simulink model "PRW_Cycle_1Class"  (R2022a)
settings: Solver=VariableStepAuto  StartTime=0.0  StopTime=simtime  RelTol=1e-3
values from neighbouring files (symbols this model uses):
  GT = SOH_p01(data_length_finish,1)    [Data_preparation.m]    (also in SimulationCycle.m = 1)
libraries: neural x35

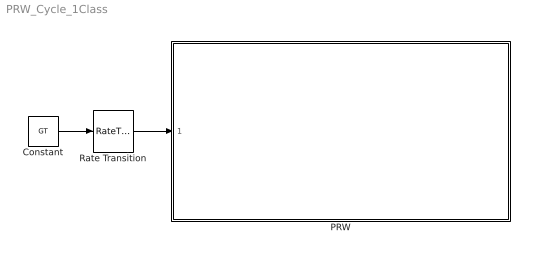
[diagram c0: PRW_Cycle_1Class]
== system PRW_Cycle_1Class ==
  Constant : Constant  Value=GT
  PRW : Subsystem
  Rate Transition : RateTransition  OutPortSampleTime=1
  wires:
  Rate Transition/1 -> PRW/1(SOH)
  Constant/1 -> Rate Transition/1

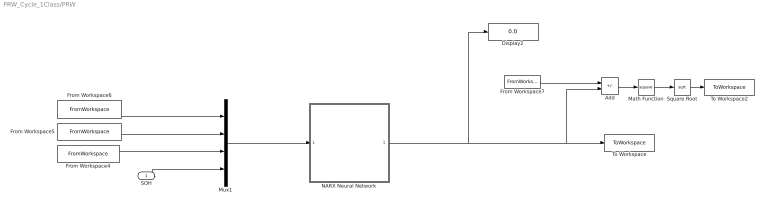
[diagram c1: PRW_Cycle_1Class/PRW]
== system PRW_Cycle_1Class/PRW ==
  SOH : Inport
  Add : Sum  Inputs=+-
  Display2 : Display
  From Workspace4 : FromWorkspace  VariableName=Temperature37
  From Workspace5 : FromWorkspace  VariableName=Voltage37  SampleTime=1
  From Workspace6 : FromWorkspace  VariableName=Current37  SampleTime=1
  From Workspace7 : FromWorkspace  VariableName=SOC_37_GT
  Math Function : Math  Operator=square
  Mux1 : Mux
  NARX Neural Network : Subsystem  mask{pi_input_1_delayed_1=[0.510586069346425031056924126460216939449310302734375;0.94022295872250705173200913122855126857757568359375;-0.58565072302558396355465220040059648454189300537109375;0.6993682659832136661037793601281009614467620849609375], ai_layer_2_delayed_1=0.999984478854660352453720406629145145416259765625}
      mask prompts: pi_input_1_delayed_1 "Preprocessed initial input 1 state at timestep 0."; ai_layer_2_delayed_1 "Initial layer 2 state at timestep 0."
      mask help: NARX Neural Network
  Square Root : Sqrt
  To Workspace : ToWorkspace  VariableName=SOC_37_pred  SaveFormat=Timeseries  SampleTime=-1
  To Workspace2 : ToWorkspace  VariableName=SOC_37_abserror  SampleTime=-1
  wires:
  From Workspace6/1 -> Mux1/1
  From Workspace5/1 -> Mux1/2
  From Workspace4/1 -> Mux1/3
  Mux1/1 -> NARX Neural Network/1(x)
  SOH/1 -> Mux1/4
  Math Function/1 -> Square Root/1
  NARX Neural Network/1(y) -> To Workspace/1, Add/2, Display2/1
  From Workspace7/1 -> Add/1
  Add/1 -> Math Function/1
  Square Root/1 -> To Workspace2/1

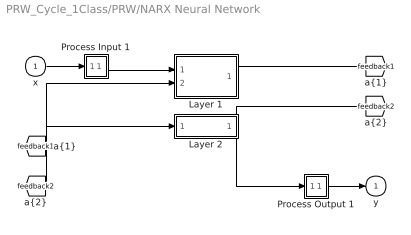
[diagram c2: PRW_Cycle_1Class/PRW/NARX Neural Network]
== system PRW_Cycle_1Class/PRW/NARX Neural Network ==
  x : Inport  PortDimensions=4  SampleTime=1
  Layer 1 : Subsystem
  Layer 2 : Subsystem
  Process Input 1 : Subsystem
  Process Output 1 : Subsystem
  y : Outport  InitialOutput=0
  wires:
  x/1 -> Process Input 1/1(x)
  Process Output 1/1(y) -> y/1
  Process Input 1/1(p) -> Layer 1/1("p{1}")
  Layer 1/1("a{1}") -> [feedback1]
  [feedback1] -> Layer 2/1("a{1} ")
  Layer 2/1("a{2}") -> [feedback2], Process Output 1/1(a)
  [feedback2] -> Layer 1/2("a{2} ")

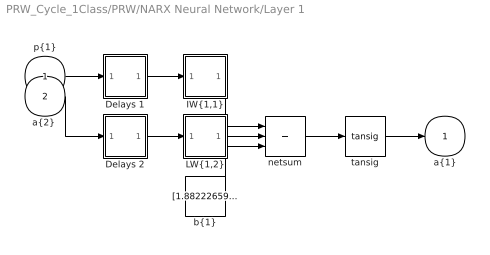
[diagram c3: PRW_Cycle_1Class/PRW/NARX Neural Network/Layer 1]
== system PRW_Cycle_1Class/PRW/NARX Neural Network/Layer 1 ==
  "p{1}" : Inport  PortDimensions=4  SampleTime=1
  "a{2} " : Inport  Port=2  PortDimensions=1  SampleTime=1
  Delays 1 : Subsystem
  Delays 2 : Subsystem
  "IW{1,1}" : Subsystem
  "LW{1,2}" : Subsystem
  "b{1}" : Constant  Value=[1.8822265945278056076261918860836885869503021240234375;-1.6332926436185550844726321884081698954105377197265625;-1.3416753095284523755736927341786213219165802001953125;0.6041072172283656893654324449016712605953216552734375;-0.1437522046735665026684358736019930802285671234130859375;-0.706093682503903696812130874604918062686920166015625;-0.32497208659573073585846714195213280618190765380859375;-0.355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
  netsum : Sum  Inputs=3  InputSameDT=on  SaturateOnIntegerOverflow=on
  tansig : neural/Transfer Functions/tansig
  "a{1}" : Outport  InitialOutput=[0;0;0;0;0;0;0;0;0;0;0;0;0;0;0]
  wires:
  "p{1}"/1 -> Delays 1/1("p{1}")
  Delays 1/1("pd{1,1}") -> "IW{1,1}"/1("pd{1,1}")
  "IW{1,1}"/1("iz{1,1}") -> netsum/1
  "a{2} "/1 -> Delays 2/1("p{1}")
  Delays 2/1("pd{1,2}") -> "LW{1,2}"/1("ad{1,2}")
  "LW{1,2}"/1("lz{1,2}") -> netsum/2
  "b{1}"/1 -> netsum/3
  netsum/1 -> tansig/1
  tansig/1 -> "a{1}"/1

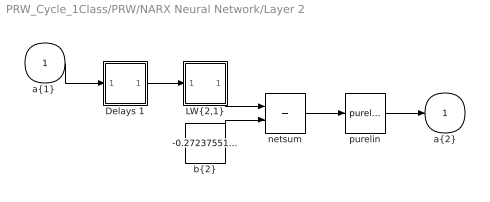
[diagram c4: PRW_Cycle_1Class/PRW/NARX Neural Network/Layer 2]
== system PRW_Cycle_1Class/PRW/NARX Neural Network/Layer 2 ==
  "a{1} " : Inport  PortDimensions=15  SampleTime=1
  Delays 1 : Subsystem
  "LW{2,1}" : Subsystem
  "b{2}" : Constant  Value=-0.272375519140338695489589326825807802379131317138671875
  netsum : Sum  Inputs=2  InputSameDT=on  SaturateOnIntegerOverflow=on
  purelin : neural/Transfer Functions/purelin
  "a{2}" : Outport  InitialOutput=0
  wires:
  "a{1} "/1 -> Delays 1/1("p{2}")
  Delays 1/1("pd{2,1}") -> "LW{2,1}"/1("ad{2,1}")
  "LW{2,1}"/1("lz{2,1}") -> netsum/1
  "b{2}"/1 -> netsum/2
  netsum/1 -> purelin/1
  purelin/1 -> "a{2}"/1

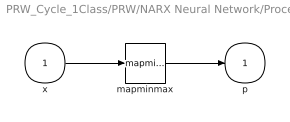
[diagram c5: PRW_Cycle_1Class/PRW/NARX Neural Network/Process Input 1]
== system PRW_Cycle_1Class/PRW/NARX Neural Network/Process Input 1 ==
  x : Inport  PortDimensions=4  SampleTime=1
  mapminmax : neural/Processing Functions/mapminmax  xmin=[-4.92400000000000037658764995285;2.50570000000000003836930773105;17.1380000000000016768808563938;0.835541218929458540110033482051]  xmax=[1.59400000000000008348877145181;4.1652000000000004575895218295;31.5220000000000020179413695587;1.02410814058582477770187324495]  ymin=-1  ymax=1
  p : Outport  PortDimensions=4  SampleTime=1
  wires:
  x/1 -> mapminmax/1
  mapminmax/1 -> p/1

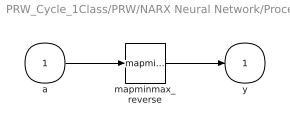
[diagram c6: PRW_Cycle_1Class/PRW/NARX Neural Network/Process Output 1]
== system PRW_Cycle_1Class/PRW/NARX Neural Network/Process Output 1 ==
  a : Inport  PortDimensions=1  SampleTime=1
  mapminmax_reverse : neural/Processing Functions/mapminmax_reverse  xmin=-4.21949321457851519659313158095e-06  xmax=1.00000776066564278643511443079  ymin=-1  ymax=1
  y : Outport  PortDimensions=1  SampleTime=1
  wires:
  a/1 -> mapminmax_reverse/1
  mapminmax_reverse/1 -> y/1

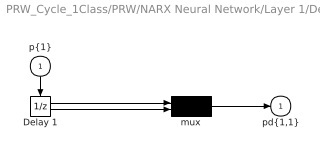
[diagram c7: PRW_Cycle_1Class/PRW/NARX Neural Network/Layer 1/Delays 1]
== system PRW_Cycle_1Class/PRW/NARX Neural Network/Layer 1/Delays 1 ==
  "p{1}" : Inport  PortDimensions=4  SampleTime=1
  Delay 1 : UnitDelay  InitialCondition=pi_input_1_delayed_1
  mux : Mux  Inputs=2
  "pd{1,1}" : Outport
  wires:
  "p{1}"/1 -> Delay 1/1, mux/1
  Delay 1/1 -> mux/2
  mux/1 -> "pd{1,1}"/1

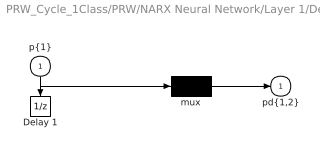
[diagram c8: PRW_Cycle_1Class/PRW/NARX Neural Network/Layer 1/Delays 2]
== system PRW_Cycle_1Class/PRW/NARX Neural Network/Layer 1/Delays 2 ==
  "p{1}" : Inport  PortDimensions=1  SampleTime=1
  Delay 1 : UnitDelay  InitialCondition=ai_layer_2_delayed_1
  mux : Mux  Inputs=1
  "pd{1,2}" : Outport
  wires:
  "p{1}"/1 -> Delay 1/1
  Delay 1/1 -> mux/1
  mux/1 -> "pd{1,2}"/1

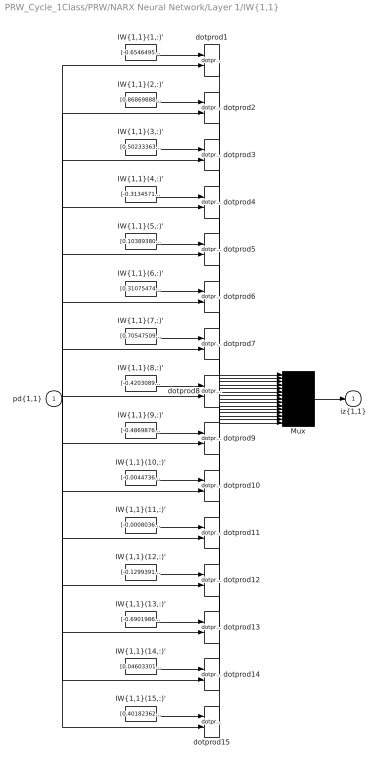
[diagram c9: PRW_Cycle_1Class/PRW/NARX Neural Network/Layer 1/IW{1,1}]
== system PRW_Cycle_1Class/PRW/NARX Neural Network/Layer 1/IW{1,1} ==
  "pd{1,1}" : Inport  PortDimensions=8  SampleTime=1
  "IW{1,1}(1,:)'" : Constant  Value=[-0.65464958479642942901222113505355082452297210693359375;-0.65337619102749877608715678434236906468868255615234375;-0.27677406513585223191142858922830782830715179443359375;0.699544740445478652191013679839670658111572265625;-0.5327508487652377056065233773551881313323974609375;0.655183920476839265489843455725349485874176025390625;0.54512357541839839836228520653094165027141571044921875;0.732399389771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
  "IW{1,1}(10,:)'" : Constant  Value=[-0.004473615007626346833091712795749117503874003887176513671875;0.037970600901949515260103140690262080170214176177978515625;0.000622190521338159062240957819511777415755204856395721435546875;-0.73937293258495884185066415739129297435283660888671875;0.006270143855257244956680207081944899982772767543792724609375;-0.0434914184436572259784270499949343502521514892578125;-0.000978375828634564905297854586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
  "IW{1,1}(11,:)'" : Constant  Value=[-0.000803688640588731575790937267100844110245816409587860107421875;0.007304655688605474032903952519291124190203845500946044921875;0.000179303297634150521529250443819591964711435139179229736328125;-0.64174790841768747373663472899352200329303741455078125;0.00110522572626375425834666099689229668001644313335418701171875;-0.0086662725370479885833585598220452084206044673919677734375;-0.0002161151422075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
  "IW{1,1}(12,:)'" : Constant  Value=[-0.1299391138224756103713986021830351091921329498291015625;-0.3108468188756159378272059257142245769500732421875;-0.301381656439640599476348370444611646234989166259765625;0.813926715557872437756259387242607772350311279296875;0.79444213433619748077063604796421714127063751220703125;-0.74333106820964023331299586061504669487476348876953125;-0.93001715117281469336063537411973811686038970947265625;0.773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
  "IW{1,1}(13,:)'" : Constant  Value=[-0.69019861384391345549005336579284630715847015380859375;0.303517311344015328078427273794659413397312164306640625;-0.11588968500930464655684914987432421185076236724853515625;0.0333233741271399541705733327034977264702320098876953125;0.34215290948315502106424901285208761692047119140625;0.719303753429601844260332654812373220920562744140625;0.1932183998067463492898099275407730601727962493896484375;0.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
  "IW{1,1}(14,:)'" : Constant  Value=[0.046033014342807855590056220762562588788568973541259765625;-0.320009483124574500845227476020227186381816864013671875;-0.0037827151657194740298761903574131792993284761905670166015625;-0.48998833707874134280046973799471743404865264892578125;-0.0559539845377299560613693074628827162086963653564453125;0.35603064580821264240029222492012195289134979248046875;0.004948006288950728380482413371055372408591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
  "IW{1,1}(15,:)'" : Constant  Value=[0.40182362320964504220910384901799261569976806640625;0.443797221498127114625020794846932403743267059326171875;0.404736354887146154712951329202041961252689361572265625;-0.5444547322933590560722905138391070067882537841796875;-0.499221102235928693158228952597710303962230682373046875;0.326541136120923447538899608844076283276081085205078125;-0.78482570856269562309392995302914641797542572021484375;0.36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
  "IW{1,1}(2,:)'" : Constant  Value=[0.86869888871761968829332545283250510692596435546875;0.72024101342312529805411713823559693992137908935546875;0.53978291332661820778326955405646003782749176025390625;1.0762178046281662968652881318121217191219329833984375;-0.5937142553320791105164744294597767293453216552734375;-0.04866153831105286819980193513401900418102741241455078125;0.028861609457539870449149788100839941762387752532958984375;0.6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
  "IW{1,1}(3,:)'" : Constant  Value=[0.502333636054542953530699378461576998233795166015625;-0.04217064256693146828691709515624097548425197601318359375;0.97775496427980745917096783159649930894374847412109375;0.0765530654322205961204161894784192554652690887451171875;-0.9206174201497259179660659356159158051013946533203125;-0.86991362119887083448332987245521508157253265380859375;-0.697857414960799449232808910892345011234283447265625;0.3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
  "IW{1,1}(4,:)'" : Constant  Value=[-0.31345714847786154688691340197692625224590301513671875;0.85034755000740480657128728125826455652713775634765625;0.56028050229703418860793817657395265996456146240234375;-0.037903152207868197332008008970660739578306674957275390625;-0.389621350223876616869489453165442682802677154541015625;-0.558085972171615818382406359887681901454925537109375;0.328888134142325483377788941652397625148296356201171875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
  "IW{1,1}(5,:)'" : Constant  Value=[0.10389380656564677074538138867865200154483318328857421875;-0.71531407808736535702820447113481350243091583251953125;-0.00881952900832292351063212976214344962500035762786865234375;-0.42724834169698355790245614116429351270198822021484375;-0.12428511357538195303273909075869596563279628753662109375;0.78620701918519320106071290865656919777393341064453125;0.012385218222176220051466977167820004979148507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
  "IW{1,1}(6,:)'" : Constant  Value=[0.31075474918349199615619227188290096819400787353515625;-0.86954687162722421600591360402177087962627410888671875;-0.227267153693776868816911473913933150470256805419921875;-0.46922022354537407107244462167727760970592498779296875;0.84939914624888890326559476307011209428310394287109375;-0.34023298555811376520097155662369914352893829345703125;-0.96089900795011995437988616686197929084300994873046875;0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
  "IW{1,1}(7,:)'" : Constant  Value=[0.70547509207102432338132302902522496879100799560546875;0.5333216507004916451251119724474847316741943359375;0.241259959791017164487669788286439143121242523193359375;0.7234565154870693515221091729472391307353973388671875;0.88144459725232271463113420395529828965663909912109375;-0.5530186873877471764870961123961023986339569091796875;-0.49338163591327732770963621078408323228359222412109375;-0.8750598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
  "IW{1,1}(8,:)'" : Constant  Value=[-0.420308996663344147659557847873657010495662689208984375;-1.00456689250621433728838383103720843791961669921875;-0.557251798636304584988465649075806140899658203125;-0.07655558877503908232764473495990387164056301116943359375;-0.77595128658275935862320693559013307094573974609375;0.6684410342356186252033012351603247225284576416015625;-0.16022457961280556215655224150395952165126800537109375;-0.580934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
  "IW{1,1}(9,:)'" : Constant  Value=[-0.486987618942922473319612208797479979693889617919921875;0.96359550467118404437627532388432882726192474365234375;-0.073130027070734737737467412443947978317737579345703125;-1.0254000463140282572993555731954984366893768310546875;-0.049334409015149995048066244862638995982706546783447265625;0.0794147500705200959369989277547574602067470550537109375;-0.2092932986342730117268473577496479265391826629638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
  Mux : Mux  Inputs=15
  dotprod{1..15} (15 alike) : neural/Weight Functions/dotprod
  "iz{1,1}" : Outport
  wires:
  "IW{1,1}(1,:)'"/1 -> dotprod1/1
  "pd{1,1}"/1 -> dotprod1/2, dotprod2/2, dotprod3/2, dotprod4/2, dotprod5/2, dotprod6/2, dotprod7/2, dotprod8/2, dotprod9/2, dotprod10/2, dotprod11/2, dotprod12/2, dotprod13/2, dotprod14/2, dotprod15/2
  dotprod1/1 -> Mux/1
  "IW{1,1}(2,:)'"/1 -> dotprod2/1
  dotprod2/1 -> Mux/2
  "IW{1,1}(3,:)'"/1 -> dotprod3/1
  dotprod3/1 -> Mux/3
  "IW{1,1}(4,:)'"/1 -> dotprod4/1
  dotprod4/1 -> Mux/4
  "IW{1,1}(5,:)'"/1 -> dotprod5/1
  dotprod5/1 -> Mux/5
  "IW{1,1}(6,:)'"/1 -> dotprod6/1
  dotprod6/1 -> Mux/6
  "IW{1,1}(7,:)'"/1 -> dotprod7/1
  dotprod7/1 -> Mux/7
  "IW{1,1}(8,:)'"/1 -> dotprod8/1
  dotprod8/1 -> Mux/8
  "IW{1,1}(9,:)'"/1 -> dotprod9/1
  dotprod9/1 -> Mux/9
  "IW{1,1}(10,:)'"/1 -> dotprod10/1
  dotprod10/1 -> Mux/10
  "IW{1,1}(11,:)'"/1 -> dotprod11/1
  dotprod11/1 -> Mux/11
  "IW{1,1}(12,:)'"/1 -> dotprod12/1
  dotprod12/1 -> Mux/12
  "IW{1,1}(13,:)'"/1 -> dotprod13/1
  dotprod13/1 -> Mux/13
  "IW{1,1}(14,:)'"/1 -> dotprod14/1
  dotprod14/1 -> Mux/14
  "IW{1,1}(15,:)'"/1 -> dotprod15/1
  dotprod15/1 -> Mux/15
  Mux/1 -> "iz{1,1}"/1

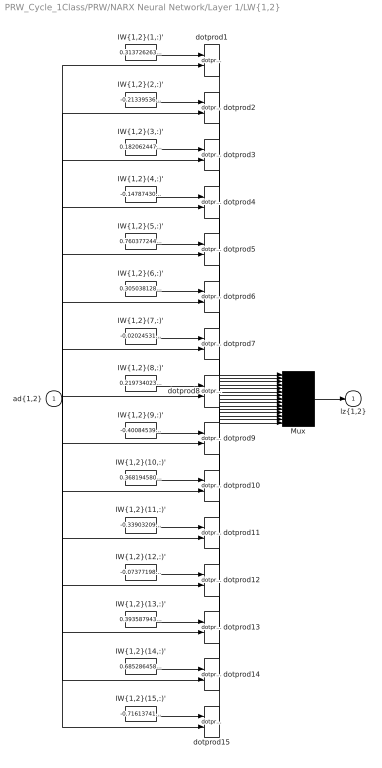
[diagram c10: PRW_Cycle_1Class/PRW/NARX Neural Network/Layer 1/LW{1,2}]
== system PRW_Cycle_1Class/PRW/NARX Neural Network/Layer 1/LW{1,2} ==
  "ad{1,2}" : Inport  PortDimensions=1  SampleTime=1
  "IW{1,2}(1,:)'" : Constant  Value=0.313726263793036863614105413944344036281108856201171875
  "IW{1,2}(10,:)'" : Constant  Value=0.368194580241390401198486870271153748035430908203125
  "IW{1,2}(11,:)'" : Constant  Value=-0.33903209028859737639294280597823671996593475341796875
  "IW{1,2}(12,:)'" : Constant  Value=-0.073771982169325178713137347585870884358882904052734375
  "IW{1,2}(13,:)'" : Constant  Value=0.39358794392944795870192820075317285954952239990234375
  "IW{1,2}(14,:)'" : Constant  Value=0.685286458039714663215136170038022100925445556640625
  "IW{1,2}(15,:)'" : Constant  Value=-0.7161374180503587982826729785301722586154937744140625
  "IW{1,2}(2,:)'" : Constant  Value=-0.213395363259064108074625210065278224647045135498046875
  "IW{1,2}(3,:)'" : Constant  Value=0.1820624470642757675165057662525214254856109619140625
  "IW{1,2}(4,:)'" : Constant  Value=-0.1478743086424599562089809978715493343770503997802734375
  "IW{1,2}(5,:)'" : Constant  Value=0.76037724464155143078158971547964029014110565185546875
  "IW{1,2}(6,:)'" : Constant  Value=0.305038128522850116031150946582783944904804229736328125
  "IW{1,2}(7,:)'" : Constant  Value=-0.02024531678997439076983511085927602834999561309814453125
  "IW{1,2}(8,:)'" : Constant  Value=0.21973402384318896363168960306211374700069427490234375
  "IW{1,2}(9,:)'" : Constant  Value=-0.400845396189503710981938411350711248815059661865234375
  Mux : Mux  Inputs=15
  dotprod{1..15} (15 alike) : neural/Weight Functions/dotprod
  "lz{1,2}" : Outport
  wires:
  "IW{1,2}(1,:)'"/1 -> dotprod1/1
  "ad{1,2}"/1 -> dotprod1/2, dotprod2/2, dotprod3/2, dotprod4/2, dotprod5/2, dotprod6/2, dotprod7/2, dotprod8/2, dotprod9/2, dotprod10/2, dotprod11/2, dotprod12/2, dotprod13/2, dotprod14/2, dotprod15/2
  dotprod1/1 -> Mux/1
  "IW{1,2}(2,:)'"/1 -> dotprod2/1
  dotprod2/1 -> Mux/2
  "IW{1,2}(3,:)'"/1 -> dotprod3/1
  dotprod3/1 -> Mux/3
  "IW{1,2}(4,:)'"/1 -> dotprod4/1
  dotprod4/1 -> Mux/4
  "IW{1,2}(5,:)'"/1 -> dotprod5/1
  dotprod5/1 -> Mux/5
  "IW{1,2}(6,:)'"/1 -> dotprod6/1
  dotprod6/1 -> Mux/6
  "IW{1,2}(7,:)'"/1 -> dotprod7/1
  dotprod7/1 -> Mux/7
  "IW{1,2}(8,:)'"/1 -> dotprod8/1
  dotprod8/1 -> Mux/8
  "IW{1,2}(9,:)'"/1 -> dotprod9/1
  dotprod9/1 -> Mux/9
  "IW{1,2}(10,:)'"/1 -> dotprod10/1
  dotprod10/1 -> Mux/10
  "IW{1,2}(11,:)'"/1 -> dotprod11/1
  dotprod11/1 -> Mux/11
  "IW{1,2}(12,:)'"/1 -> dotprod12/1
  dotprod12/1 -> Mux/12
  "IW{1,2}(13,:)'"/1 -> dotprod13/1
  dotprod13/1 -> Mux/13
  "IW{1,2}(14,:)'"/1 -> dotprod14/1
  dotprod14/1 -> Mux/14
  "IW{1,2}(15,:)'"/1 -> dotprod15/1
  dotprod15/1 -> Mux/15
  Mux/1 -> "lz{1,2}"/1

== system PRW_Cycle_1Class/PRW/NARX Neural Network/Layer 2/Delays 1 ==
  "p{2}" : Inport  PortDimensions=15  SampleTime=1
  mux : Mux  Inputs=1
  "pd{2,1}" : Outport
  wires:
  "p{2}"/1 -> mux/1
  mux/1 -> "pd{2,1}"/1

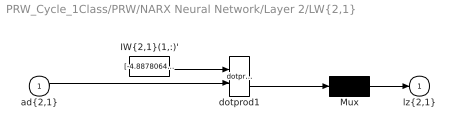
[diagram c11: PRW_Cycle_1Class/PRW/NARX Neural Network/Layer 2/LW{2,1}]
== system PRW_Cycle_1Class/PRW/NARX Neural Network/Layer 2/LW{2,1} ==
  "ad{2,1}" : Inport  PortDimensions=15  SampleTime=1
  "IW{2,1}(1,:)'" : Constant  Value=[-4.887806461353221866572571485676235170103609561920166015625e-05;-3.889267473351513330730166995152785602840594947338104248046875e-05;2.300146907736462680341658904037416277787997387349605560302734375e-05;0.0001665013286308004666382009961722587831900455057621002197265625;0.034971929797273981765926009757095016539096832275390625;7.729981660706192189767664568744720554605009965598583221435546875e-06;6.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
  Mux : Mux  Inputs=1
  dotprod1 : neural/Weight Functions/dotprod
  "lz{2,1}" : Outport
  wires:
  "IW{2,1}(1,:)'"/1 -> dotprod1/1
  "ad{2,1}"/1 -> dotprod1/2
  dotprod1/1 -> Mux/1
  Mux/1 -> "lz{2,1}"/1
